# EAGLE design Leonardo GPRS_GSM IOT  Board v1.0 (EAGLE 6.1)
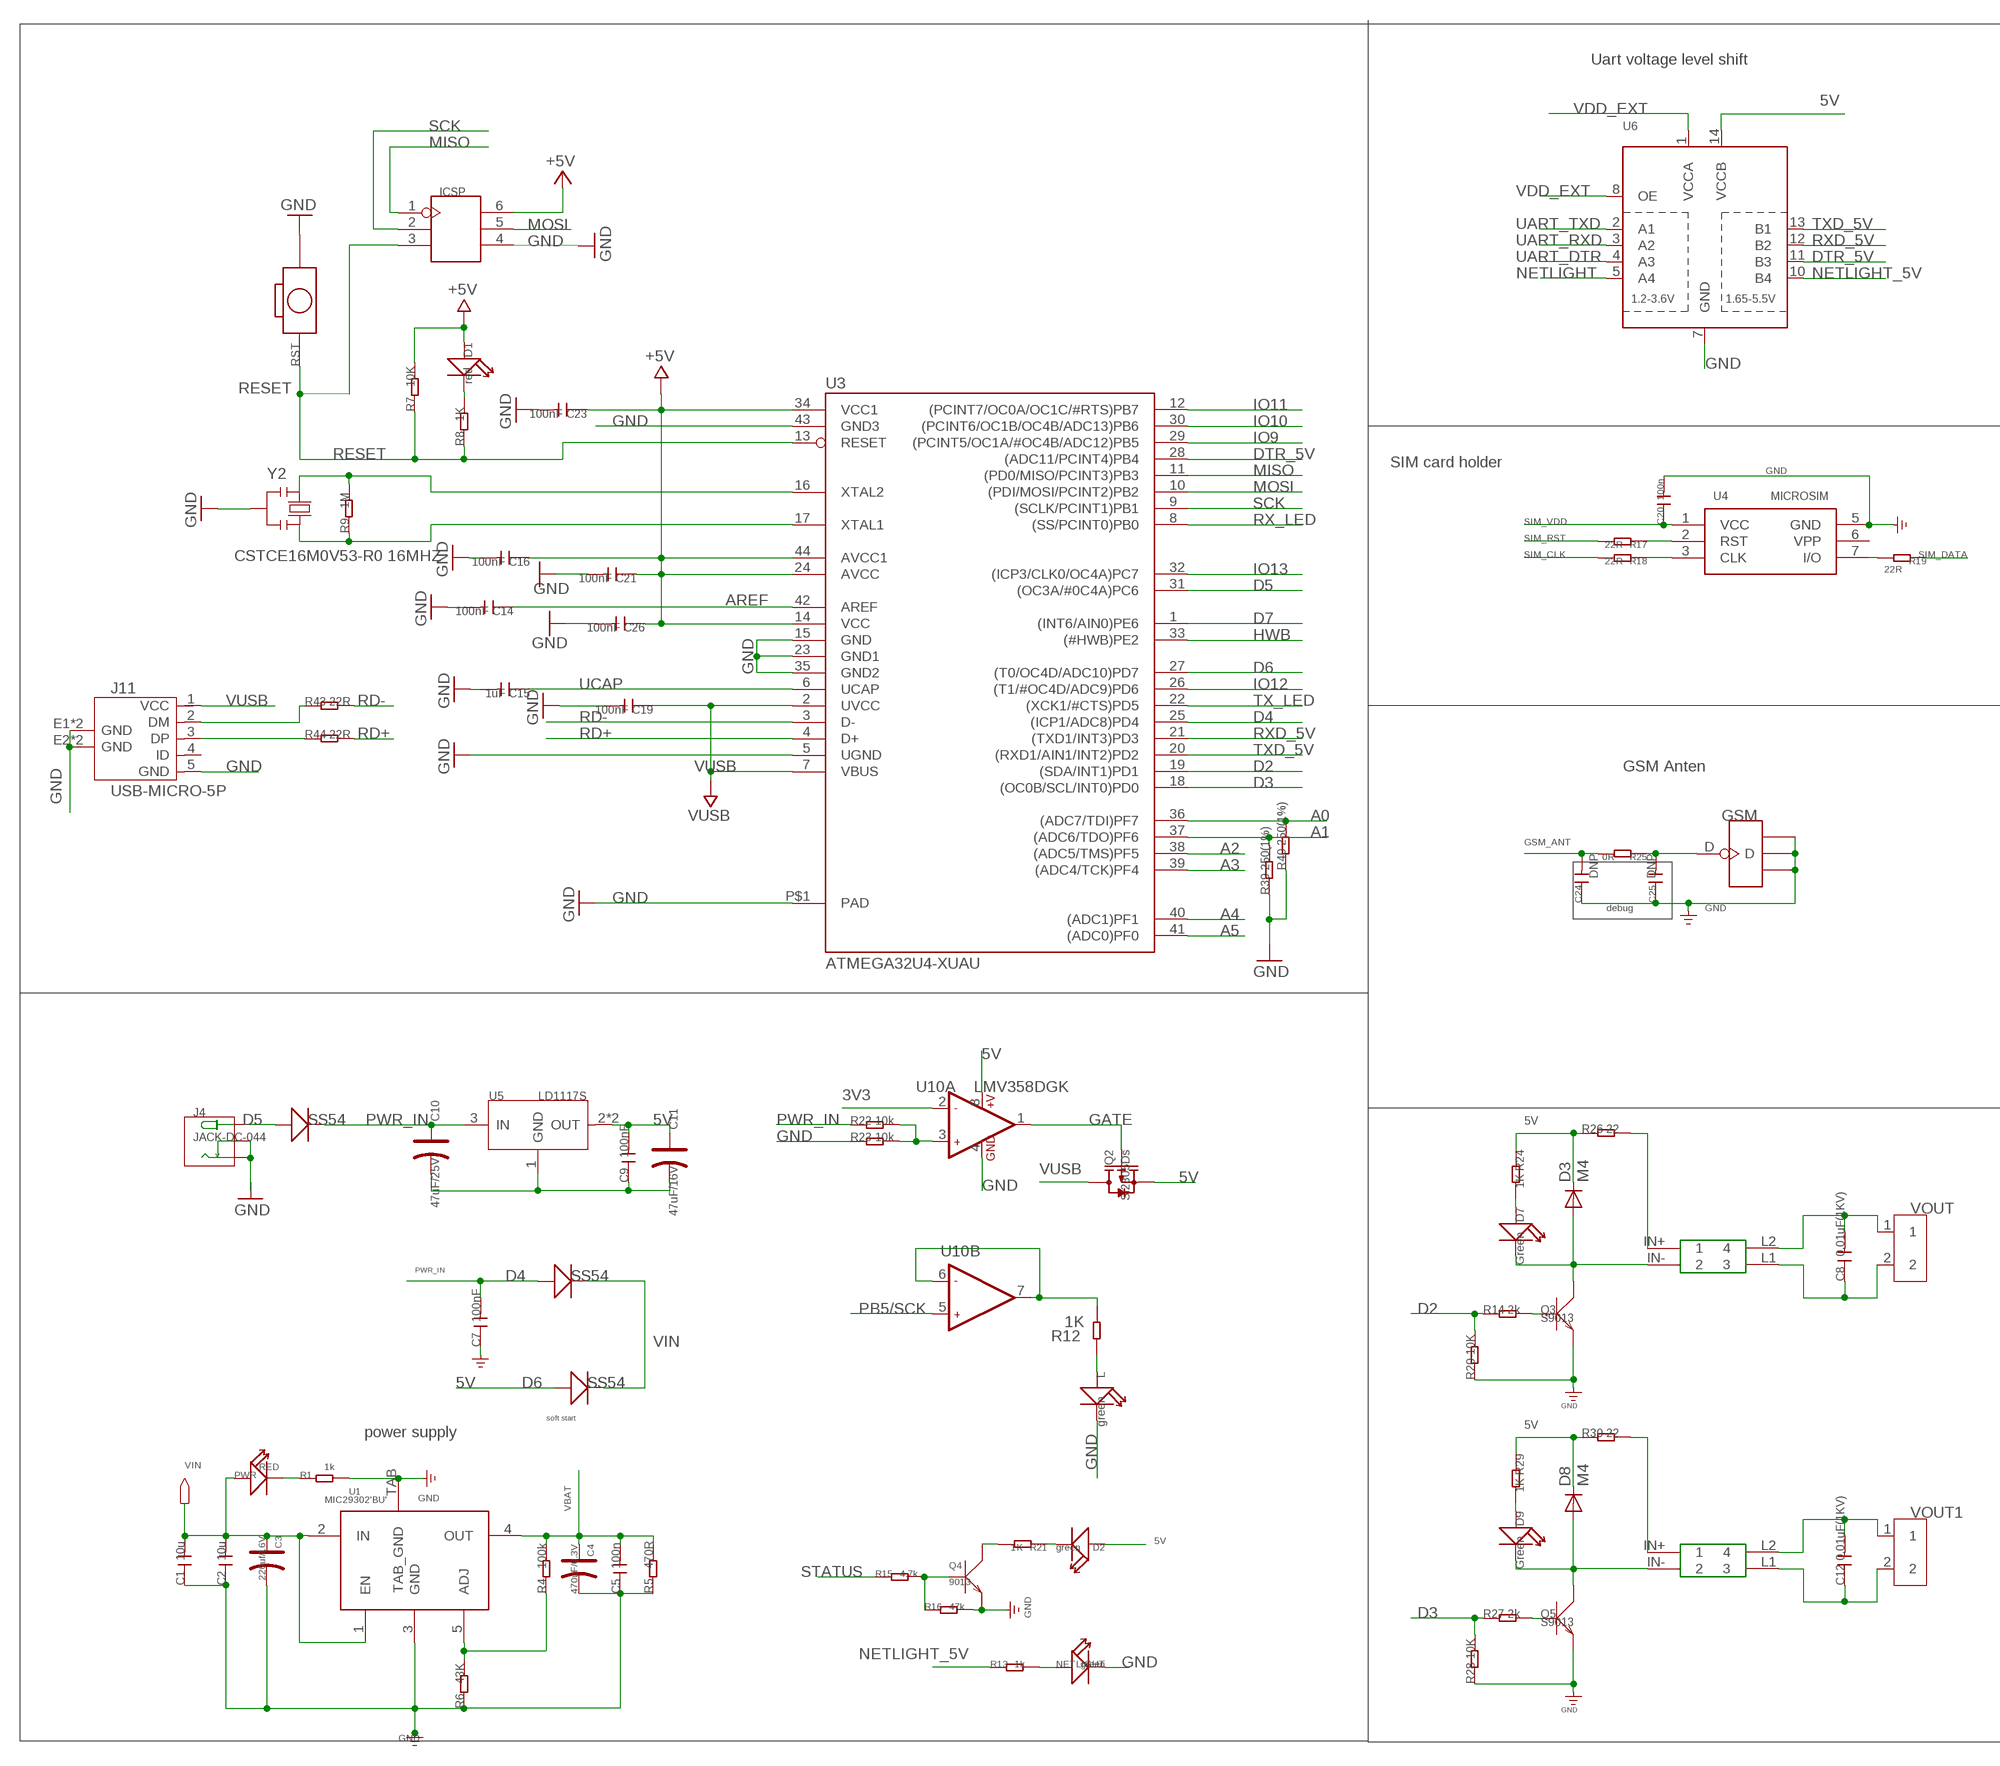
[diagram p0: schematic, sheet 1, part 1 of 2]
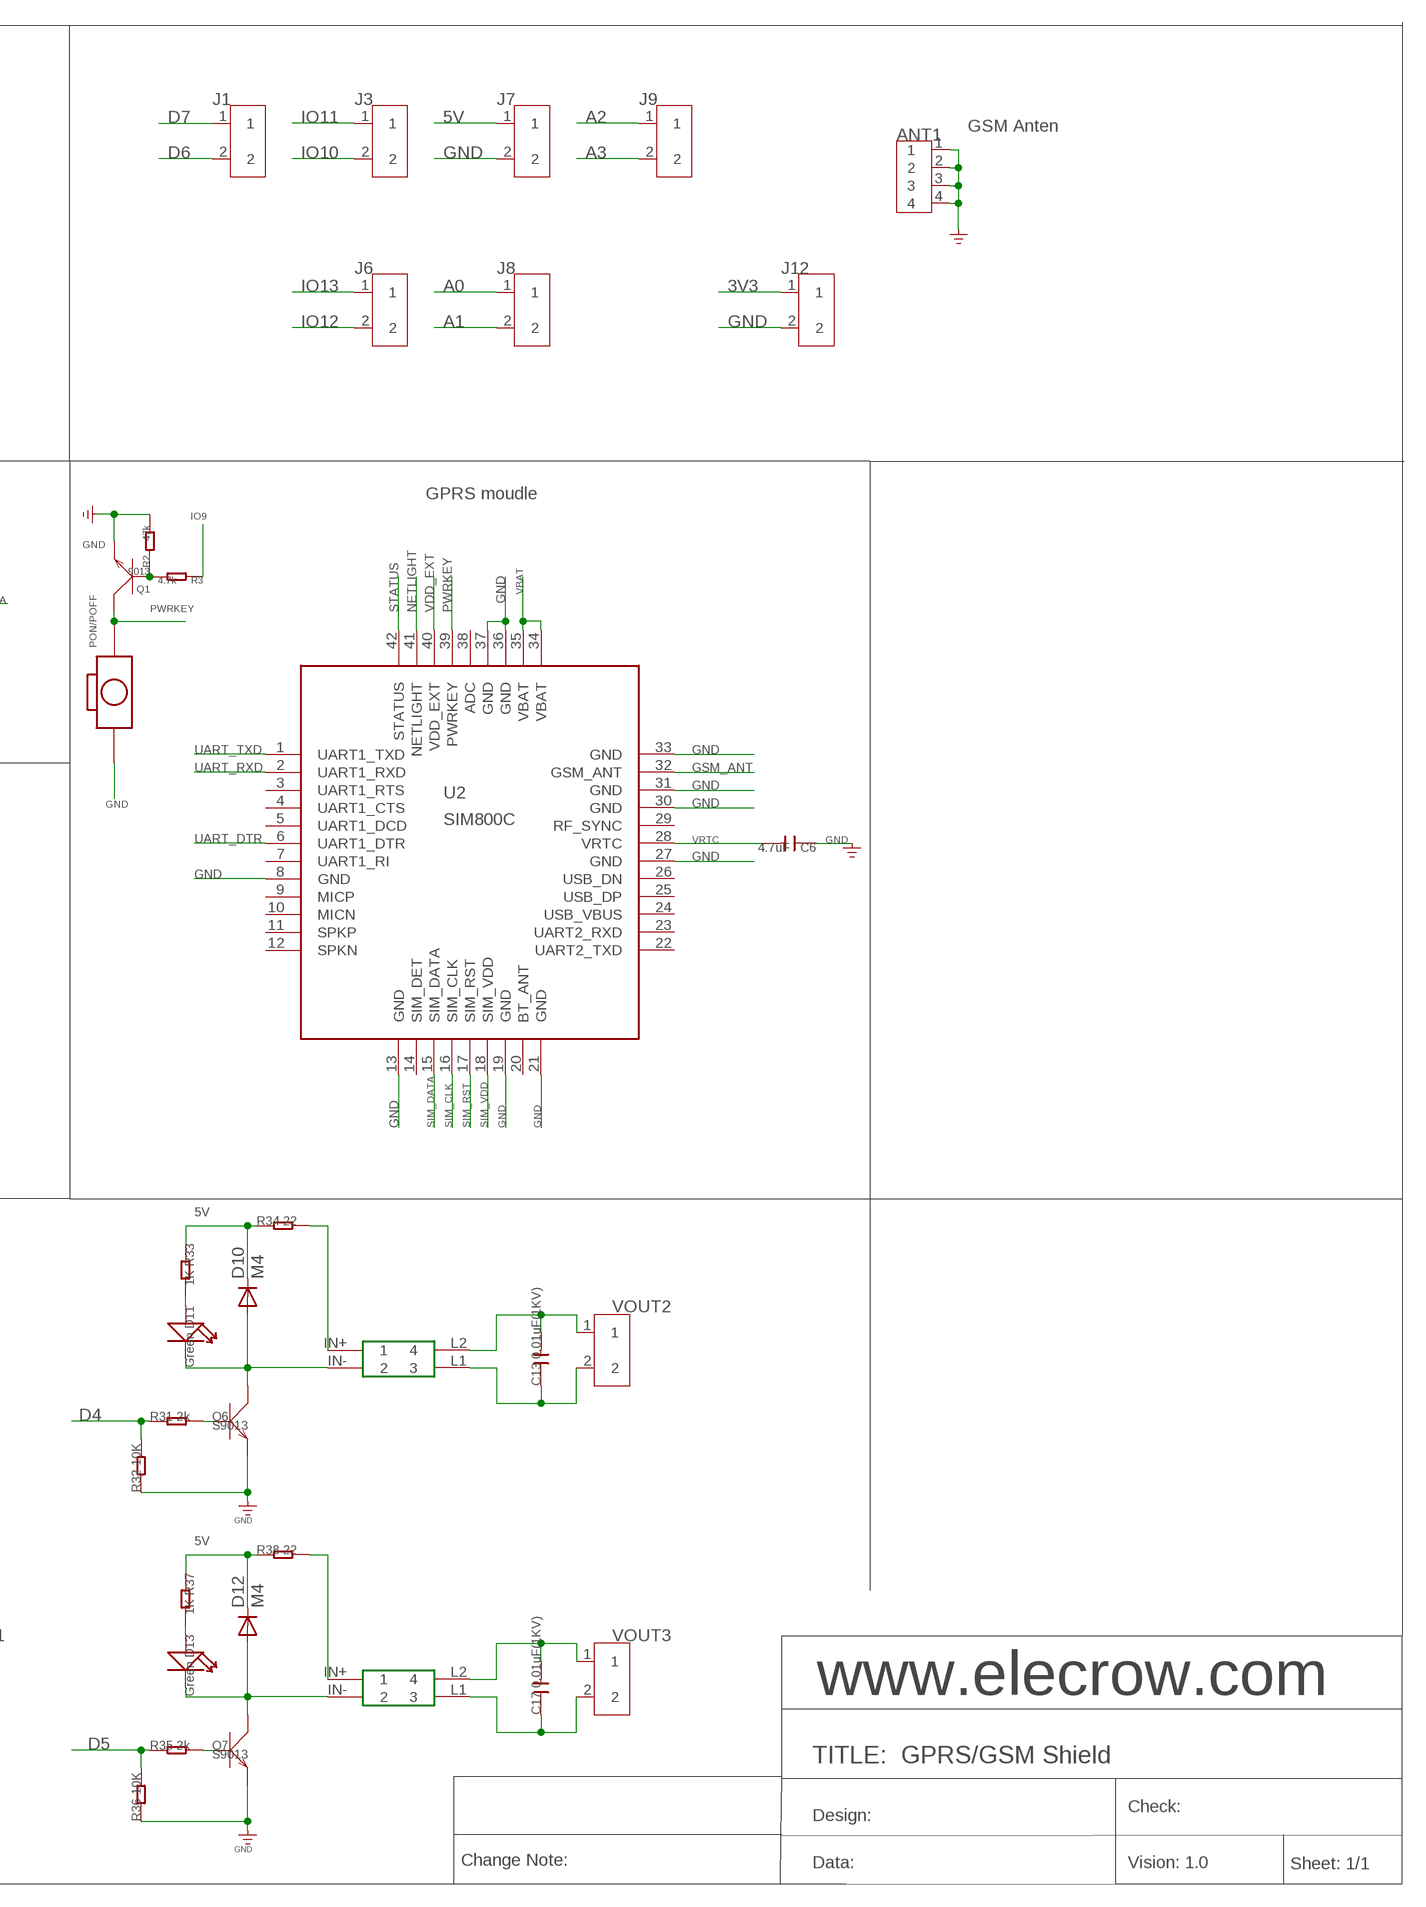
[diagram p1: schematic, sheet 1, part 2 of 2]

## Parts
ANT1  ANTENNA-SMA-IPX  [SMA-TO-IPX]
C1  10u  C-0603  [C0603]
C2  10u  C-0603  [C0603]
C3  220uf/16V  006-CAP_AVX_D  [AVX_D]
C4  470uF/6.3V  006-CAP_AVX_D  [AVX_D]
C5  100n  C-0603  [C0603]
C6  4.7uF  C-0805  [C0805]
C7  100nF  C-0603  [C0603]
C8  0.01uF(1KV)  C-1206  [C1206]
C9  100nF  C-0603  [C0603]
C10  47uF/25V  CAP-AVX-C  [AVX-C]
C11  47uF/16V  CAP-AVX-A  [AVX-A]
C12  0.01uF(1KV)  C-1206  [C1206]
C13  0.01uF(1KV)  C-1206  [C1206]
C14  100nF  C-0603  [C0603]
C15  1uF  C-0603  [C0603]
C16  100nF  C-0603  [C0603]
C17  0.01uF(1KV)  C-1206  [C1206]
C19  100nF  C-0603  [C0603]
C20  100n  C-0603  [C0603]
C21  100nF  C-0603  [C0603]
C23  100nF  C-0603  [C0603]
C24  DNP  C-0402  [C0402]
C25  DNP  C-0402  [C0402]
C26  100nF  C-0603  [C0603]
D1  red  LED'0603'  [LED-0603]
D2  green  LED'0603'  [LED-0603]
D3  M4  DIODE-DO-214AC  [DO-214AC]
D4  SS54  D'MBRS240LT3'  [SMB]
D5  SS54  D'MBRS240LT3'  [SMB]
D6  SS54  D'MBRS240LT3'  [SMB]
D7  Green  LED'0603'  [LED-0603]
D8  M4  DIODE-DO-214AC  [DO-214AC]
D9  Green  LED'0603'  [LED-0603]
D10  M4  DIODE-DO-214AC  [DO-214AC]
D11  Green  LED'0603'  [LED-0603]
D12  M4  DIODE-DO-214AC  [DO-214AC]
D13  Green  LED'0603'  [LED-0603]
GSM  ANTENNA-U-FL  [4P-U-FL]
ICSP  HEADER-2X3P-2.0  [2X3P-2.0]
J1  SCREW-TERMINAL-2P'5.0'  [2P-5.0]
J3  SCREW-TERMINAL-2P'5.0'  [2P-5.0]
J4  JACK-DC-044  [DC-404]
J6  SCREW-TERMINAL-2P'5.0'  [2P-5.0]
J7  SCREW-TERMINAL-2P'5.0'  [2P-5.0]
J8  SCREW-TERMINAL-2P'5.0'  [2P-5.0]
J9  SCREW-TERMINAL-2P'5.0'  [2P-5.0]
J11  USB-MICRO-5P  [MICRO-USB-5P]
J12  SCREW-TERMINAL-2P'5.0'  [2P-5.0]
L  green  LED'0603'  [LED-0603]
NETLIGHT  green  LED'0603'  [LED-0603]
PON/POFF  BOTTON_1_DP  [BTN_5.0_RST]
PWR  RED  007-LED0603  [D0603]
Q1  9013  TRANSISTOR-NPN-SOT23  [SOT23]
Q2  Si2305Ds  MOSFET-P'SI2323CDS/SI2305DS<BR>'  [SOT23@2]
Q3  S9013  TRANSISTOR-NPN-SOT23  [SOT23]
Q4  9013  TRANSISTOR-NPN-SOT23  [SOT23]
Q5  S9013  TRANSISTOR-NPN-SOT23  [SOT23]
Q6  S9013  TRANSISTOR-NPN-SOT23  [SOT23]
Q7  S9013  TRANSISTOR-NPN-SOT23  [SOT23]
R1  1k  R-0603  [R0603]
R2  47k  R-0603  [R0603]
R3  4.7k  R-0603  [R0603]
R4  100k  R-0603  [R0603]
R5  470R  R-0603  [R0603]
R6  43K  R-0603  [R0603]
R7  10K  R-0603  [R0603]
R8  1K  R-0603  [R0603]
R9  1M  R-0603  [R0603]
R12  1K  R-0603  [R0603]
R13  1k  R-0603  [R0603]
R14  2k  R-0603  [R0603]
R15  4.7k  R-0603  [R0603]
R16  47k  R-0603  [R0603]
R17  22R  R-0603  [R0603]
R18  22R  R-0603  [R0603]
R19  22R  R-0603  [R0603]
R20  10K  R-0603  [R0603]
R21  1K  R-0603  [R0603]
R22  10k  R-0603  [R0603]
R23  10k  R-0603  [R0603]
R24  1K  R-0603  [R0603]
R25  0R  R-0402  [R0402]
R26  22  R-0603  [R0603]
R27  2k  R-0603  [R0603]
R28  10K  R-0603  [R0603]
R29  1K  R-0603  [R0603]
R30  22  R-0603  [R0603]
R31  2k  R-0603  [R0603]
R32  10K  R-0603  [R0603]
R33  1K  R-0603  [R0603]
R34  22  R-0603  [R0603]
R35  2k  R-0603  [R0603]
R36  10K  R-0603  [R0603]
R37  1K  R-0603  [R0603]
R38  22  R-0603  [R0603]
R39  250(1%)  R-0603  [R0603]
R40  250(1%)  R-0603  [R0603]
R43  22R  R-0603  [R0603]
R44  22R  R-0603  [R0603]
RST  BOTTON-2P-90D  [2P-7.62X3.56-90D]
U1  MIC29302'BU'  [TO-263]
U2  SIM800C  [SIM800C]
U3  ATMEGA32U4-XUAU  [TQFP44-PAD]
U4  MICROSIM  [MICROSIM]
U5  LD1117S  [SOT-223]
U6  TXB0104PWR  [TSSOP14]
U10  LMV358DGK  [MSOP8]
U$5  G3MB-202(RELAY)  [G3MB-202(RELAY)]
U$8  G3MB-202(RELAY)  [G3MB-202(RELAY)]
U$10  G3MB-202(RELAY)  [G3MB-202(RELAY)]
U$12  G3MB-202(RELAY)  [G3MB-202(RELAY)]
VOUT  SCREW-TERMINAL-2P'5.0'  [2P-5.0]
VOUT1  SCREW-TERMINAL-2P'5.0'  [2P-5.0]
VOUT2  SCREW-TERMINAL-2P'5.0'  [2P-5.0]
VOUT3  SCREW-TERMINAL-2P'5.0'  [2P-5.0]
Y2  CSTCE16M0V53-R0 16MHZ  RESONATORMU  [RESONATOR]

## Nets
3V3: J12.1 U10.2(A:-IN1)
5V: C9.2 C11.+ C16.1 C21.1 C23.1 C26.1 D2.+ D3.C D6.+ D8.C D10.C D12.C ICSP.6 J7.1 Q2.2(S) R24.1 R26.1 R29.1 R30.1 R33.1 R34.1 R37.1 R38.1 U3.14(VCC) U3.24(AVCC) U3.34(VCC1) U3.44(AVCC1) U5.2(OUT) U5.TER(OUT) U6.14(VCCB) U10.8(A:+V) ; supply symbol labelled +5V
+5V: D1.+ R7.2
A0: J8.1 R40.2 U3.36((ADC7/TDI)PF7)
A1: J8.2 R39.2 U3.37((ADC6/TDO)PF6)
A2: J9.1 U3.38((ADC5/TMS)PF5)
A3: J9.2 U3.39((ADC4/TCK)PF4)
A4: U3.40((ADC1)PF1)
A5: U3.41((ADC0)PF0)
AREF: C14.1 U3.42(AREF)
D2: R14.1 R20.2 U3.19((SDA/INT1)PD1)
D3: R27.1 R28.2 U3.18((OC0B/SCL/INT0)PD0)
D4: R31.1 R32.2 U3.25((ICP1/ADC8)PD4)
D5: R35.1 R36.2 U3.31((OC3A/#0C4A)PC6)
D6: J1.2 U3.27((T0/OC4D/ADC10)PD7)
D7: J1.1 U3.1((INT6/AIN0)PE6)
D+1: J11.3(DP) R44.1
D-1: J11.2(DM) R43.1
DTR_5V: U3.28((ADC11/PCINT4)PB4) U6.11(B3)
GATE: Q2.1(G) U10.1(A:OUT1)
GND: ANT1.1 ANT1.2 ANT1.3 ANT1.4 C1.1 C2.1 C3.- C4.- C5.1 C6.1 C7.1 C9.1 C10.- C11.- C14.2 C15.2 C16.2 C19.2 C20.2 C21.2 C23.2 C24.1 C25.1 C26.2 GSM.GND1 GSM.GND2 GSM.GND3 ICSP.4 J4.- J4.CDN J7.2 J11.5(GND) J11.E1(GND) J11.E2(GND) J11.P1(GND) J11.P2(GND) J12.2 L.- NETLIGHT.- PON/POFF.P$1 Q1.2(E) Q3.2(E) Q4.2(E) Q5.2(E) Q6.2(E) Q7.2(E) R1.2 R2.2 R5.1 R6.1 R16.2 R20.1 R23.1 R28.1 R32.1 R36.1 R39.1 R40.1 RST.P$2 U1.3(GND) U1.TAB(TAB_GND) U2.8(GND) U2.13(GND) U2.19(GND) U2.21(GND) U2.27(GND) U2.30(GND) U2.31(GND) U2.33(GND) U2.36(GND) U2.37(GND) U3.5(UGND) U3.15(GND) U3.23(GND1) U3.35(GND2) U3.43(GND3) U3.P$1(PAD) U4.5(GND) U5.1(GND) U6.7(GND) U10.4(A:GND) Y2.2
GSM_ANT: C24.2 R25.2 U2.32(GSM_ANT)
HWB: U3.33((#HWB)PE2)
IO9: R3.1 U3.29((PCINT5/OC1A/#OC4B/ADC12)PB5)
IO10: J3.2 U3.30((PCINT6/OC1B/OC4B/ADC13)PB6)
IO11: J3.1 U3.12((PCINT7/OC0A/OC1C/#RTS)PB7)
IO12: J6.2 U3.26((T1/#OC4D/ADC9)PD6)
IO13: J6.1 U3.32((ICP3/CLK0/OC4A)PC7)
MISO: ICSP.1 U3.11((PD0/MISO/PCINT3)PB3)
MOSI: ICSP.5 U3.10((PDI/MOSI/PCINT2)PB2)
N$1: R19.2 U4.7(I/O)
N$2: R4.1 R6.2 U1.5(ADJ)
N$3: Q3.1(B) R14.2
N$4: D5.+ J4.+
N$5: R18.1 U4.3(CLK)
N$6: R17.1 U4.2(RST)
N$7: NETLIGHT.+ R13.2
N$8: D3.A D7.- Q3.3(C) U$5.IN-
N$9: L.+ R12.2
N$10: Q6.1(B) R31.2
N$11: R12.1 U10.6(B:-IN2) U10.7(B:OUT2)
N$12: D7.+ R24.2
N$13: D10.A D11.- Q6.3(C) U$10.IN-
N$14: R22.2 R23.2 U10.3(A:+IN1)
N$15: D1.- R8.2
N$16: Q4.3(C) R21.2
N$17: D2.- R21.1
N$18: Q4.1(B) R15.2 R16.1
N$19: R26.2 U$5.IN+
N$20: C8.2 U$5.L2 VOUT.1
N$21: C8.1 U$5.L1 VOUT.2
N$22: Q5.1(B) R27.2
N$23: D8.A D9.- Q5.3(C) U$8.IN-
N$24: D9.+ R29.2
N$25: C25.2 GSM.D R25.1
N$26: R30.2 U$8.IN+
N$27: C12.2 U$8.L2 VOUT1.1
N$28: C12.1 U$8.L1 VOUT1.2
N$29: D11.+ R33.2
N$30: R34.2 U$10.IN+
N$31: C13.2 U$10.L2 VOUT2.1
N$32: C13.1 U$10.L1 VOUT2.2
N$33: Q7.1(B) R35.2
N$34: D12.A D13.- Q7.3(C) U$12.IN-
N$35: D13.+ R37.2
N$36: Q1.1(B) R2.1 R3.2
N$37: R38.2 U$12.IN+
N$38: C17.2 U$12.L2 VOUT3.1
N$39: C17.1 U$12.L1 VOUT3.2
N$53: PWR.- R1.1
NETLIGHT: U2.41(NETLIGHT) U6.5(A4)
NETLIGHT_5V: R13.1 U6.10(B4)
PB5/SCK: U10.5(B:+IN2)
PWR_IN: C7.2 C10.+ D4.+ D5.- R22.1 U5.3(IN)
PWRKEY: PON/POFF.P$2 Q1.3(C) U2.39(PWRKEY)
RD+: R44.2 U3.4(D+)
RD-: R43.2 U3.3(D-)
RESET: ICSP.3 R7.1 R8.1 RST.P$1 U3.13(RESET)
RX_LED: U3.8((SS/PCINT0)PB0)
RXD_5V: U3.21((TXD1/INT3)PD3) U6.12(B2)
SCK: ICSP.2 U3.9((SCLK/PCINT1)PB1)
SIM_CLK: R18.2 U2.16(SIM_CLK)
SIM_DATA: R19.1 U2.15(SIM_DATA)
SIM_RST: R17.2 U2.17(SIM_RST)
SIM_VDD: C20.1 U2.18(SIM_VDD) U4.1(VCC)
STATUS: R15.1 U2.42(STATUS)
TX_LED: U3.22((XCK1/#CTS)PD5)
TXD_5V: U3.20((RXD1/AIN1/INT2)PD2) U6.13(B1)
UART_DTR: U2.6(UART1_DTR) U6.4(A3)
UART_RXD: U2.2(UART1_RXD) U6.3(A2)
UART_TXD: U2.1(UART1_TXD) U6.2(A1)
UCAP: C15.1 U3.6(UCAP)
VBAT: C4.+ C5.2 R4.2 R5.2 U1.4(OUT) U2.34(VBAT) U2.35(VBAT)
VDD_EXT: U2.40(VDD_EXT) U6.1(VCCA) U6.8(OE)
VIN: C1.2 C2.2 C3.+ D4.- D6.- PWR.+ U1.1(EN) U1.2(IN)
VRTC: C6.2 U2.28(VRTC)
VUSB: C19.1 J11.1(VCC) Q2.3(D) U3.2(UVCC) U3.7(VBUS)
XTAL3: R9.2 U3.16(XTAL2) Y2.1
XTAL4: R9.1 U3.17(XTAL1) Y2.3
Unconnected: J11.4(ID) U2.3(UART1_RTS) U2.4(UART1_CTS) U2.5(UART1_DCD) U2.7(UART1_RI) U2.9(MICP) U2.10(MICN) U2.11(SPKP) U2.12(SPKN) U2.14(SIM_DET) U2.20(BT_ANT) U2.22(UART2_TXD) U2.23(UART2_RXD) U2.24(USB_VBUS) U2.25(USB_DP) U2.26(USB_DN) U2.29(RF_SYNC) U2.38(ADC) U4.6(VPP)

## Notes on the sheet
- Uart voltage level shift
- GSM Anten
- GPRS moudle
- SIM card holder
- GSM Anten
- debug
- soft start
- power supply
- www.elecrow.com
- TITLE:  GPRS/GSM Shield
- Check:
- Design:
- Change Note: | Data: | Vision: 1.0 | Sheet: 1/1

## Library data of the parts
ANT1 = Connector:ANTENNA-SMA-IPX
C1 C2 C5-C9 C12-C17 C19-C21 C23-C26 = Discrete:C*: Ceramic Capacitors
C3 C4 = Discrete:006-CAP*: Electrolytic Capacitors,Tantalum Capacitors and Super Capacitors
C10 C11 = Discrete:CAP*: Electrolytic Capacitors,Tantalum Capacitors and Super Capacitors
D1 D2 D7 D9 D11 D13 L NETLIGHT = Discrete:LED*
D3 D8 D10 D12 = diode:DIODE-: DIODE
D4-D6 = Discrete:D*
GSM = Connector:ANTENNA-U-FL
ICSP = Connector:HEADER-2X3P
J1 J3 J6-J9 J12 VOUT VOUT1-VOUT3 = Connector:SCREW-TERMINAL-2P
J4 = Connector:JACK-DC-044
J11 = Connector:USB-MICRO-5P
PON/POFF = CPT_SMD:BOTTON_1
PWR = Discrete:007-LED*
Q1 Q3-Q7 = Discrete:TRANSISTOR-NPN*: NPN audion
Q2 = Discrete:MOSFET-P
R1-R9 R12-R40 R43 R44 = Discrete:R*
RST = Discrete:BOTTON-2P
U1 = ICs_v54:MIC29302
U2 = moudle:SIM800C
U3 = SmartPrj:ATMEGA32U4-XU
U4 = Connector:MICROSIM
U5 = IC:LD1117: Low Drop Fixed And Adjustable Positive Voltage Regulators http://www.datasheetcatalog.org/datasheet/SGSThomsonMicroelectronics/mXuqtqv.pdf
U6 = adafruit:TXB0104PWR: 4-Bit Bi-Directional Level Shifter 1.2V-3.6V (VCCA) to 1.65V-5.5V (VCCB) bi-directional level shifter with auto direction sensing. Max data rate - VCCA 1.8V: 20Mbps (50ns), VCCA 3.3V: 100Mbps (10ns) Digikey: 296-21929-1-ND
U10 = IC:LMV358: General purpose LOW Voltage, Rail-to-Rail Output Amplifiers http://www.fairchildsemi.com/ds/LM/LMV358.pdf
U$5 U$8 U$10 U$12 = G3MB-202(relay):G3MB-202(RELAY)
Y2 = SmartPrj:RESONATOR

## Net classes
0 default: width 0.152 mm, drill 0.152 mm, clearance 0.152 mm
3 usbvcc: width 0.508 mm, drill 0.61 mm, clearance 0.254 mm
4 aref: width 0.254 mm, drill 0.61 mm, clearance 0.254 mm

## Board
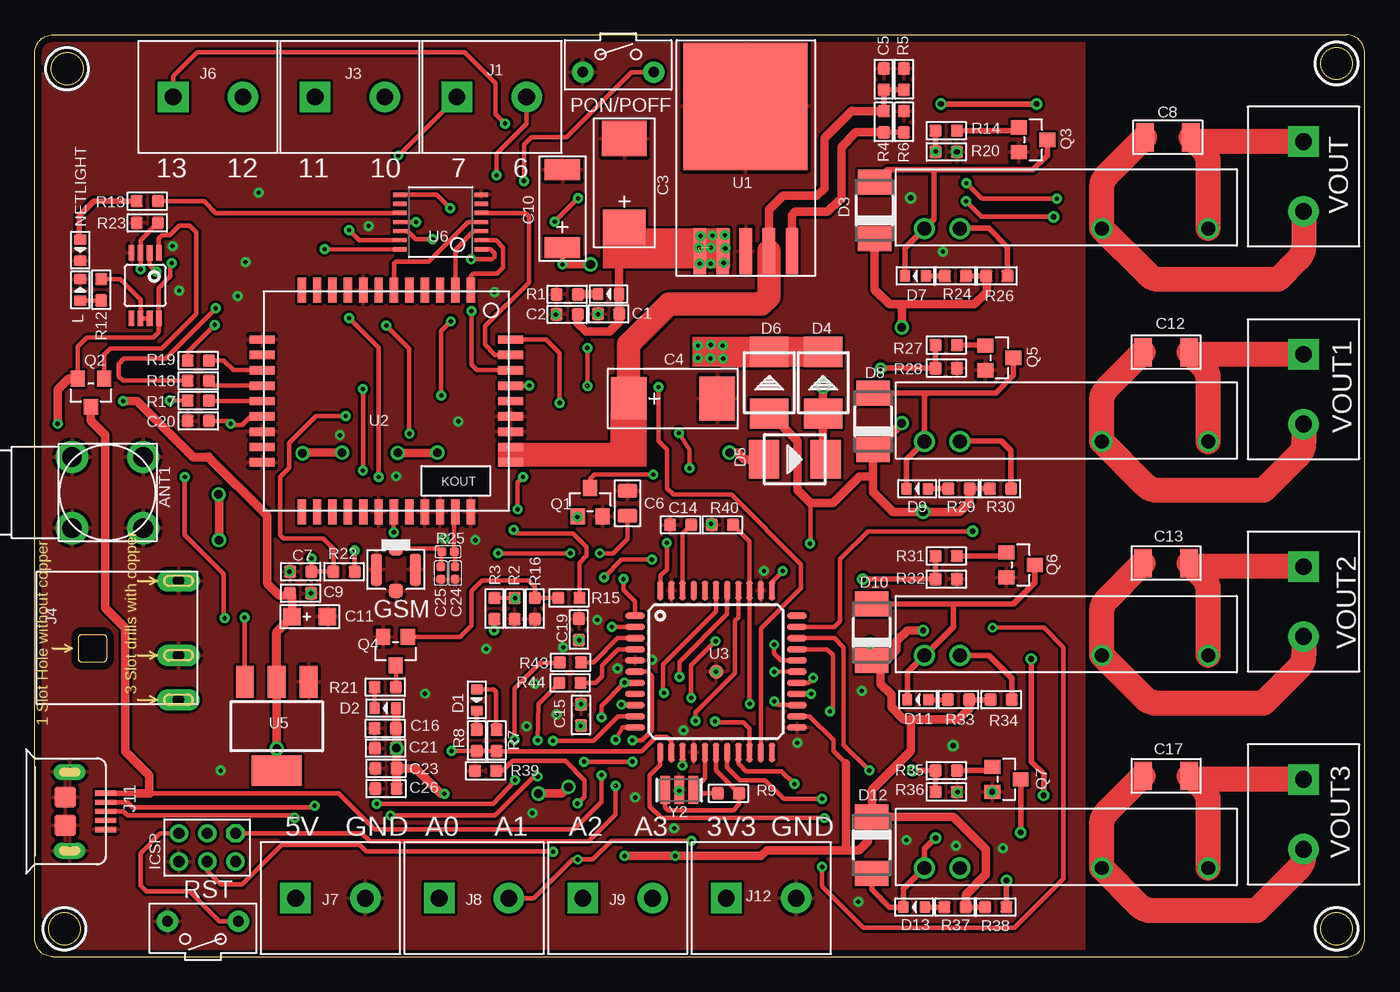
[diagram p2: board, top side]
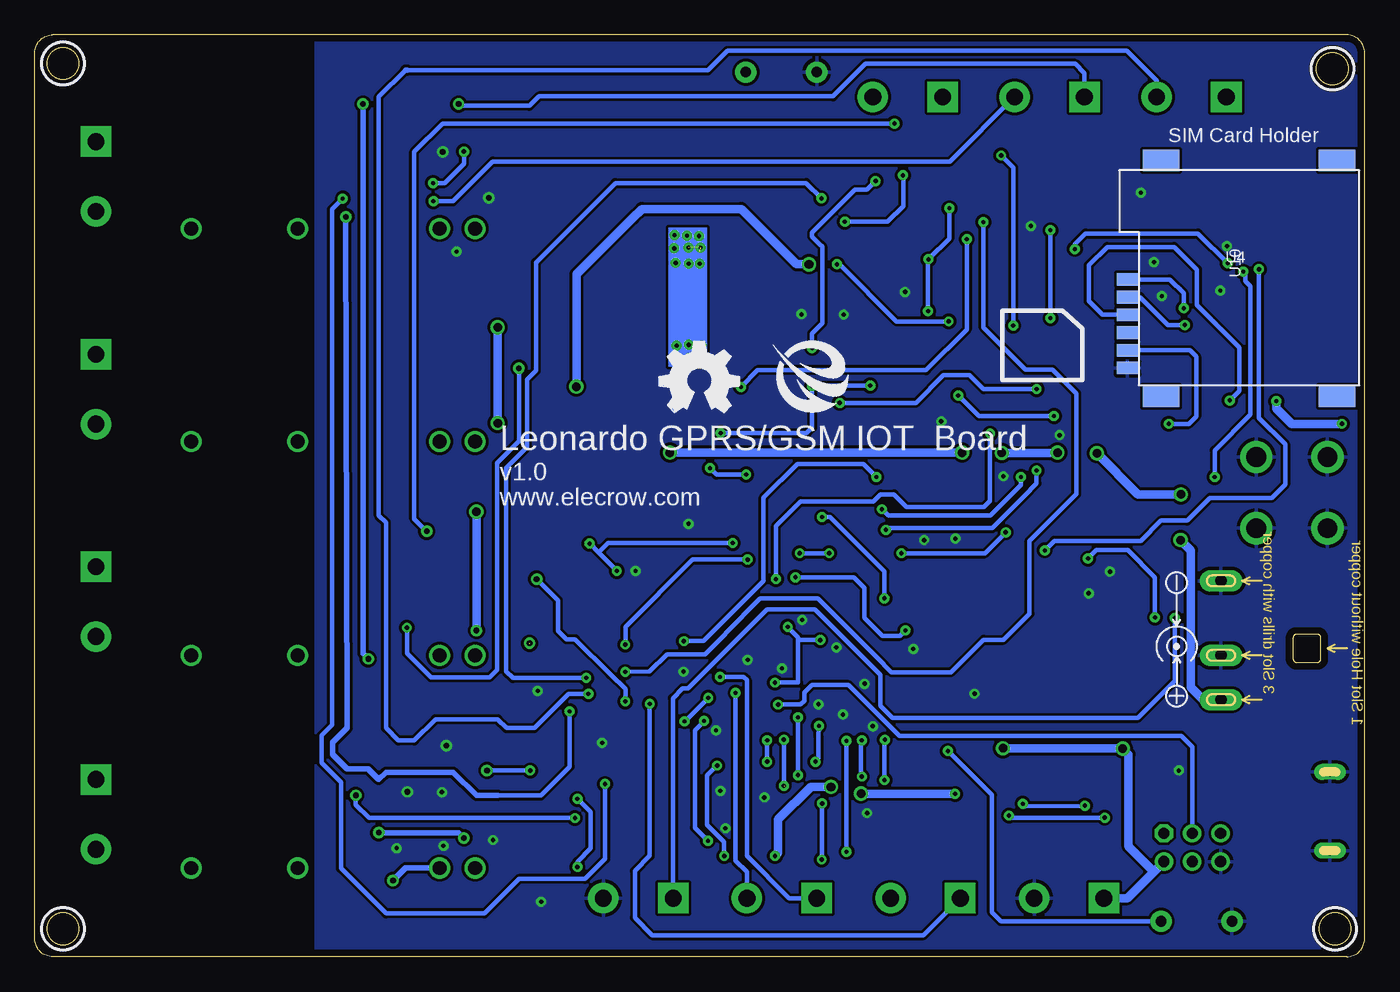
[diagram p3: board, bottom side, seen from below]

Size 95.25 x 66.04 mm. Coordinates in mm from the lower left corner, seen from the top.
Outline: 1.27,0 93.98,0 arc90 95.25,1.27 95.25,64.77 arc90 93.98,66.04 1.27,66.04 arc90 0,64.77 0,1.27 arc90 1.27,0
Outline: circle at 2.13,2 radius 1.14
Outline: circle at 2.13,2 radius 1.14
Outline: circle at 93.24,64 radius 1.14
Outline: circle at 93.24,64 radius 1.14
Outline: circle at 2.31,63.62 radius 1.14
Outline: circle at 2.31,63.62 radius 1.14
Outline: circle at 93.24,2 radius 1.14
Outline: circle at 93.24,2 radius 1.14
Copper layers (1*16): Top 0.035mm / dielectric 1.5mm / Bottom 0.035mm
Design rules: minimum track width 10mil, minimum drill 12mil, track to track 8mil, track to pad 8mil, pad to pad 8mil, via to via 8mil, smd to smd 0mil, copper to edge 20mil, drill to drill 8mil, minimum pad ring 10mil, minimum via ring 8mil, stop-mask expansion 4mil, vias tented up to drill 100mil, thermal gap 10mil
tRestrict: area 0.6,0.5 to 3.7,3.5; area 91.7,62.5 to 94.8,65.5; area 0.8,62.1 to 3.8,65.1; area 91.7,0.5 to 94.8,3.5; 1 lines
bRestrict: area 0.6,0.5 to 3.7,3.5; area 91.7,62.5 to 94.8,65.5; area 0.8,62.1 to 3.8,65.1; area 91.7,0.5 to 94.8,3.5

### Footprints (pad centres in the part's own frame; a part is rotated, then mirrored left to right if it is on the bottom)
SMA-TO-IPX = drill 1.4 pad 2.3: 1 -2.55,2.55; 2 2.55,2.55; 3 2.55,-2.55; 4 -2.55,-2.55
C0603 = smd 0.889 x 0.889: 1 -0.762,0; 2 0.762,0
AVX_D = smd 2.54 x 3.048: + -3.175,0 | smd 2.54 x 3.175: - 3.175,0
C0805 = smd 1.016 x 1.397: 1 -0.889,0; 2 0.889,0
C1206 = smd 1.27 x 2.032: 1 -1.651,0; 2 1.651,0
AVX-C = smd 1.524 x 2.54: + -2.794,0; - 2.794,0
AVX-A = smd 1.27 x 1.27: + -1.27,0; - 1.27,0
C0402 = smd 0.635 x 0.635: 1 -0.445,0; 2 0.445,0
LED-0603 = smd 0.762 x 0.889: + -0.762,0; - 0.762,0
DO-214AC = smd 1.8 x 2.4: A 2.025,0; C -2.025,0
SMB = smd 2.159 x 2.743: + -2.21,0; - 2.21,0
4P-U-FL = smd 1.016 x 1.016: D -1.524,0; GND3 1.524,0 | smd 2.286 x 0.762: GND1 0,1.397; GND2 0,-1.397
2X3P-2.0 = drill 0.813 pad 1.27 octagon: 1 -1.016,2.032 | drill 0.813 pad 1.27: 2 -1.016,0; 3 -1.016,-2.032; 4 1.016,-2.032; 5 1.016,0; 6 1.016,2.032
2P-5.0 = drill 1.2 pad 2.184 square: 1 0,0 | drill 1.2 pad 2.184: 2 5,0
DC-404 = drill 0.813 pad 1.524 long: + 3.175,10.16; - -5.334,10.16; CDN 0,10.16
MICRO-USB-5P = smd 0.38 x 1.52: 1 -1.3,0; 2 -0.65,0; 3 0,0; 4 0.65,0; 5 1.3,0 | smd 1.524 x 1.524: E1 -1.016,-2.921; E2 1.016,-2.921 | drill 0.635 pad 1.143 long: P1 -2.819,-2.591; P2 2.819,-2.591
BTN_5.0_RST = drill 0.762 pad 1.524: P$1 0,2.54; P$2 0,-2.54
D0603 = smd 0.762 x 0.889: + -0.762,0; - 0.762,0
SOT23 = smd 1.016 x 1.143: 1 -0.889,-1.016; 2 0.889,-1.016; 3 0,1.016
SOT23@2 = smd 1.016 x 1.143: 1 -0.95,-1.016; 2 0.95,-1.016; 3 0,1.016
R0603 = smd 0.889 x 0.889: 1 -0.762,0; 2 0.762,0
R0402 = smd 0.635 x 0.635: 1 -0.445,0; 2 0.445,0
2P-7.62X3.56-90D = drill 0.762 pad 1.524: P$1 0,2.54; P$2 0,-2.54
TO-263 = smd 3.302 x 0.889: 1 3.302,-3.302; 2 3.302,-1.651; 3 3.302,0; 4 3.302,1.651; 5 3.302,3.302 | smd 9.12 x 8.89: TAB -7.071,-0.03
SIM800C = smd 1.8 x 0.6: 1 -7.95,6.05; 2 -7.95,4.95; 3 -7.95,3.85; 4 -7.95,2.75; 5 -7.95,1.65; 6 -7.95,0.55; 7 -7.95,-0.55; 8 -7.95,-1.65; 9 -7.95,-2.75; 10 -7.95,-3.85; 11 -7.95,-4.95; 12 -7.95,-6.05; 22 7.95,-6.05; 23 7.95,-4.95; 24 7.95,-3.85; 25 7.95,-2.75; 26 7.95,-1.65; 27 7.95,-0.55; 28 7.95,0.55; 29 7.95,1.65; 30 7.95,2.75; 31 7.95,3.85; 32 7.95,4.95; 33 7.95,6.05 | smd 0.6 x 1.8: 13 -4.4,-8.9; 14 -3.3,-8.9; 15 -2.2,-8.9; 16 -1.1,-8.9; 17 0,-8.9; 18 1.1,-8.9; 19 2.2,-8.9; 20 3.3,-8.9; 21 4.4,-8.9; 34 4.4,8.9; 35 3.3,8.9; 36 2.2,8.9; 37 1.1,8.9; 38 0,8.9; 39 -1.1,8.9; 40 -2.2,8.9; 41 -3.3,8.9; 42 -4.4,8.9
TQFP44-PAD = smd 1.4 x 0.45: 1 -5.8,4; 2 -5.8,3.2; 3 -5.8,2.4; 4 -5.8,1.6; 5 -5.8,0.8; 6 -5.8,0; 7 -5.8,-0.8; 8 -5.8,-1.6; 9 -5.8,-2.4; 10 -5.8,-3.2; 11 -5.8,-4; 23 5.8,-4; 24 5.8,-3.2; 25 5.8,-2.4; 26 5.8,-1.6; 27 5.8,-0.8; 28 5.8,0; 29 5.8,0.8; 30 5.8,1.6; 31 5.8,2.4; 32 5.8,3.2; 33 5.8,4 | smd 0.45 x 1.4: 12 -4,-5.8; 13 -3.2,-5.8; 14 -2.4,-5.8; 15 -1.6,-5.8; 16 -0.8,-5.8; 17 0,-5.8; 18 0.8,-5.8; 19 1.6,-5.8; 20 2.4,-5.8; 21 3.2,-5.8; 22 4,-5.8; 34 4,5.8; 35 3.2,5.8; 36 2.4,5.8; 37 1.6,5.8; 38 0.8,5.8; 39 0,5.8; 40 -0.8,5.8; 41 -1.6,5.8; 42 -2.4,5.8; 43 -3.2,5.8; 44 -4,5.8 | smd 1 x 1: P$1 0,0
MICROSIM = smd 1.5 x 0.9: 1 -0.8,2.5; 2 -0.8,5.04; 3 -0.8,7.58; 5 -0.8,1.23; 6 -0.8,3.77; 7 -0.8,6.31 | smd 2.61 x 1.56: P$1 1.6,-0.8; P$2 14.2,-0.8; P$3 14.2,16.1; P$4 1.6,16.1
SOT-223 = smd 1.27 x 2.286: 1 -2.286,-3.175; 2 0,-3.175; 3 2.286,-3.175 | smd 3.556 x 2.159: TER 0,3.175
TSSOP14 = smd 0.305 x 0.991: 1 -1.95,-2.918; 2 -1.3,-2.918; 3 -0.65,-2.918; 4 0,-2.918; 5 0.65,-2.918; 6 1.3,-2.918; 7 1.95,-2.918; 8 1.95,2.918; 9 1.3,2.918; 10 0.65,2.918; 11 0,2.918; 12 -0.65,2.918; 13 -1.3,2.918; 14 -1.95,2.918
MSOP8 = smd 0.4 x 1.1: 1 -0.975,-2.35; 2 -0.325,-2.35; 3 0.325,-2.35; 4 0.975,-2.35; 5 0.975,2.35; 6 0.325,2.35; 7 -0.325,2.35; 8 -0.975,2.35
G3MB-202(RELAY) = drill 1: IN+ -7.62,2.54; IN- -10.16,2.54; L1 2.54,2.54; L2 10.16,2.54
RESONATOR = smd 0.7 x 2: 1 -1,0; 2 0,0; 3 1,0

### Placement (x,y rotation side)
ANT1  5.21,33.25 270 top
C1  41.1,46.05 0 top
C2  38.13,46.02 0 top
C3  42.23,55.44 90 top
C4  45.71,39.99 0 top
C5  60.81,62.87 270 top
C6  42.44,32.49 270 top
C7  19.05,27.58 0 top
C8  81.15,58.7 0 top
C9  19.02,26.04 180 top
C10  37.8,53.59 90 top
C11  19.68,24.36 0 top
C12  81.03,43.31 0 top
C13  81.03,28.19 0 top
C14  46.25,30.94 180 top
C15  39.12,17.32 90 top
C16  25.1,16.36 180 top
C17  81.03,12.95 0 top
C19  38.96,23.44 90 top
C20  11.71,38.39 180 top
C21  25.12,14.94 180 top
C23  25.15,13.49 180 top
C24  30.1,27.48 90 top
C25  29.08,27.48 90 top
C26  25.15,12.04 180 top
D1  31.65,18.39 270 top
D2  25.1,17.81 180 top
D3  60.15,53.47 90 top
D4  56.46,41.12 90 top
D5  54.43,35.64 0 top
D6  52.6,41.12 90 top
D7  63.07,48.77 180 top
D8  60.05,38.35 90 top
D9  63.2,33.53 180 top
D10  59.94,23.24 90 top
D11  63.25,18.41 180 top
D12  59.94,8 270 top
D13  62.99,3.56 180 top
GSM  25.86,27.74 270 top
ICSP  12.34,7.82 270 top
J1  30.23,61.59 0 top
J3  20.07,61.59 0 top
J4  0.13,21.59 270 top
J6  9.91,61.59 0 top
J7  18.67,4.19 0 top
J8  28.96,4.19 0 top
J9  39.24,4.19 0 top
J11  5.08,10.41 270 top
J12  49.53,4.19 0 top
L  3.25,47.78 90 top
LOGO2  LOGO-OSHW-FILLX0200-NT  [OSHW_FILLX200_NOTEXT]  50.5,38.99 0 bottom
NETLIGHT  3.25,50.62 270 top
PON/POFF  41.78,63.37 90 top
PWR  41.09,47.47 180 top
Q1  39.78,32.56 0 top
Q2  4.01,40.41 180 top
Q3  71.5,58.52 270 top
Q4  25.83,21.89 180 top
Q5  69.09,42.9 270 top
Q6  70.61,28.07 270 top
Q7  69.6,12.7 270 top
R1  38.13,47.46 180 top
R2  34.37,24.94 270 top
R3  32.92,24.94 90 top
R4  60.81,59.82 90 top
R5  62.26,62.87 270 top
R6  62.26,59.82 270 top
R7  33.07,15.49 90 top
R8  31.65,15.49 90 top
R9  49.68,11.71 180 top
R12  4.75,47.78 270 top
R13  8.05,54.13 180 top
R14  65.28,59.18 0 top
R15  38.25,25.7 180 top
R16  35.81,24.94 270 top
R17  11.71,39.84 0 top
R18  11.71,41.26 0 top
R19  11.71,42.71 180 top
R20  65.28,57.66 180 top
R21  25.1,19.3 0 top
R22  22.15,27.58 0 top
R23  8.05,52.58 0 top
R24  65.94,48.77 180 top
R25  29.59,29.01 0 top
R26  68.91,48.77 0 top
R27  65.28,43.81 0 top
R28  65.28,42.16 180 top
R29  66.19,33.53 180 top
R30  69.16,33.53 0 top
R31  65.28,28.7 0 top
R32  65.28,27.05 180 top
R33  66.17,18.41 180 top
R34  69.22,18.41 0 top
R35  65.28,13.34 0 top
R36  65.28,11.81 180 top
R37  65.91,3.56 180 top
R38  68.83,3.56 0 top
R39  32.28,13.31 0 top
R40  49.25,30.94 0 top
R43  38.35,21.08 0 top
R44  38.33,19.61 0 top
RST  12.04,2.54 270 top
U1  50.93,53.85 270 top
U2  25.17,39.81 270 top
U3  48.79,20.42 0 top
U4  16.18,40.94 0 bottom
U5  17.32,16.51 180 top
U6  29.06,52.63 90 top
U10  7.9,48.08 180 top
U$1  [ELECROW-NEW]  42.42,38.99 0 bottom
U$5  73.88,49.63 0 top
U$8  73.88,34.37 0 top
U$10  73.88,19.05 0 top
U$12  73.88,3.81 0 top
VOUT  90.88,58.39 270 top
VOUT1  90.88,43.15 270 top
VOUT2  90.88,27.94 270 top
VOUT3  90.88,12.7 270 top
Y2  46.15,11.94 180 top

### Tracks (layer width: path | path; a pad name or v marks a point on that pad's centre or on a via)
3V3  (via drill 0.3)
  Top 0.305: U10.2 8.22,49.53 v8.69,49.07 | v10.74,34.37 10.74,30.2 13.54,27.41 13.54,24.31 v13.59,24.26
  Bottom 0.305: v13.59,24.26 13.59,19.76 16.23,17.12 33.83,17.12 34.7,17.98 34.7,20.19 39.37,24.87 42.82,24.87 48.46,19.23 48.84,19.23 49.55,18.52 49.55,4.22 J12.1 | v8.69,49.07 8.53,48.92 8.53,48.41 8.18,48.06 8.18,38.84 10.74,36.27 v10.74,34.37
5V  (via drill 0.3, 0.41, 0.61)  (1 unrouted)
  Top 0.254: 59.69,10.16 D12.C
  Top 0.305: 25.91,14.91 C21.1 | 25.91,16.31 C16.1 | v20.75,50.7 U6.14 | v9.8,49.68 9.7,49.58 9.7,48.74 8.87,47.91 U10.8 8.87,44.74 8.48,44.35 3.71,44.35 3.06,43.7 Q2.2 2.44,41.43 | U3.24 55.5,17.22 57.2,15.52 57.2,14.76 58.12,13.84 | U3.14 46.39,13.7 v46.38,13.69 | D6.+ 52.65,38.91 | 60.05,34.39 60.07,34.42 | 52.81,26.23 U3.34 52.79,26.86 v53.57,27.64 | 55.55,32.49 55.55,29.62 v55.52,29.59 | 18.41,25.88 C9.2 18.11,25.88 | 1.65,38.2 v1.63,38.18 | v45.26,29.64 45.26,27.74 44.83,27.3 44.83,26.26 U3.44
  Top 0.406: R24.1 R26.1 68.2,48.72 | R30.1 R29.1 66.93,33.5 | D8.C 60.2,36.33 | D10.C 59.94,21.34 61.09,21.34 | R37.1 R38.1 | R33.1 R34.1 | D12.C | 60.58,20.57 59.94,21.21 D10.C | v59.82,22.45 59.82,21.34 D10.C | 62.74,16.89 62.87,17.02
  Top 0.61: D3.C 60.15,47.8 61.21,46.74 62.1,46.74 | 62.1,46.74 67.31,46.74 68.2,47.62 68.2,48.72 | D8.C 60.05,34.39 | 60.05,34.39 60.05,33.3 61.47,31.88 v63.63,31.88 66.22,31.88 66.93,32.59 66.93,33.5 | 60.2,36.33 v62.1,38.23 | v62.1,45.09 62.1,46.74 | R37.1 66.68,4.45 68.12,5.89 68.12,7.7 65.79,10.03 D12.C 59.94,11.94 62.74,14.73 62.74,16.89 | R33.1 66.93,17.78 66.17,17.02 62.87,17.02 62.23,17.02 61.34,17.91 61.34,18.8 60.58,19.56 60.58,20.57 | v63.63,23.37 62.48,23.37 61.72,22.61 61.72,21.97 61.09,21.34 | C23.1 25.91,14.91 v25.91,14.94 25.91,16.31 | C16.1 D2.+ | U5.TER v17.32,14.91 U5.2 | C26.1 C23.1 | v36.07,11.68 37.74,11.68 v38.23,12.17 | v42.24,7.21 v45.87,7.21 52.02,7.21 52.43,7.62 58.17,7.62 | 59.69,10.16 59.69,8.28 59.03,7.62 58.17,7.62 | 52.65,38.91 54.61,36.96 54.61,33.43 55.55,32.49 57.15,32.49 59.05,34.39 60.05,34.39 | C11.+ 18.41,25.88 | 11.33,35.81 7.34,39.8 v6.33,39.8 | 2.44,41.43 1.65,40.64 1.65,38.2 | 18.11,25.88 17.5,25.88 16.64,26.75 16.64,31.6 | v29.34,11.66 29.08,11.66 27.25,13.49 C23.1 | 58.12,13.84 58.12,7.67 58.17,7.62
  Top 0.66: U5.2 17.32,23.27 C11.+ | 16.64,31.6 12.42,35.81 11.33,35.81
  Bottom 0.305: 59.79,22.48 59.84,22.43 | 36.04,11.66 v36.07,11.68 | v45.87,7.21 45.87,8.23 47.09,9.45 47.09,12.98 v46.38,13.69 | v53.57,27.64 53.59,27.64 53.59,27.69 54.86,28.96 | v20.75,50.7 20.75,51.05 19.99,51.82 11.94,51.82 v9.8,49.68 | v45.26,29.64 54.18,29.64 54.86,28.96 | 54.86,28.96 55.5,29.59 v55.52,29.59
  Bottom 0.61: v62.1,38.23 v62.1,45.09 | v63.63,23.37 v63.63,31.88 | v25.91,14.94 v17.32,14.91 16.92,14.5 16.92,7.9 15.11,6.1 14.4,6.81 ICSP.6 16.99,4.19 J7.1 | v29.34,11.66 36.04,11.66 | v38.23,12.17 39.67,12.17 42.01,9.83 42.01,7.44 v42.24,7.21 | v6.33,39.8 6.33,39.27 5.23,38.18 v1.63,38.18
+5V
  Top 0.305: D1.+ 32.87,19.15 33.05,18.97 33.05,16.28 R7.2
A0  (via drill 0.3)
  Top 0.305: R40.2 51.19,29.76 U3.36 51.19,18.12 v51.21,18.11
  Bottom 0.305: J8.1 31.6,1.55 51.03,1.55 52.27,2.79 52.27,6.15 51.21,7.21 v51.21,18.11
A1  (via drill 0.3)
  Top 0.305: J8.2 35.74,4.19 38.51,6.96 v38.89,6.96 39.95,6.96 41.3,8.31 v47.04,8.31 | 38.86,10.92 38.86,10.95 | 38.86,10.95 v38.86,10.97 | 38.86,10.95 39.37,11.46 39.37,12.65 38,14.02 34.21,14.02 33.5,13.31 R39.2 | U3.37 50.39,24.31 50.16,24.08 50.16,20.34 47.32,17.5 v47.32,16.89
  Bottom 0.305: v47.32,16.89 47.32,16.87 47.98,16.2 47.98,9.25 v47.04,8.31 | v38.86,10.97 38.86,6.99 v38.89,6.96
A2  (via drill 0.3)
  Top 0.305: U3.38 49.59,24.55 46.18,21.13 v46.18,20.04
  Bottom 0.305: v46.18,20.04 44.48,20.04 44.25,19.81 44.25,7.21 41.22,4.19 J9.1
A3  (via drill 0.3)
  Top 0.305: U3.39 48.79,24.74 44.98,20.93 45.01,20.9 45.01,18.95 v45.06,18.9
  Bottom 0.305: v45.06,18.9 45.06,6.88 44.24,6.07 J9.2
AREF
  Top 0.305: U3.42 46.39,30.32 C14.1
D2  (via drill 0.3)
  Top 0.305: U3.19 50.39,13.84 50.95,13.28 53.49,13.28 v54.41,12.37 | v73.2,54.3 67.84,54.3 v66.73,55.42 | R20.2 v64.52,57.68
  Top 0.406: R20.2 R14.1
  Bottom 0.305: v54.41,12.37 54.41,7.01 55.85,5.56 60.58,5.56 63.04,3.1 70.1,3.1 73.33,6.33 73.33,12.5 74.73,13.89 74.73,15.85 73.97,16.61 73.97,53.54 v73.2,54.3 | v66.73,55.42 65.91,55.42 64.52,56.82 R20.2 64.54,57.68 v64.52,57.68
D3  (via drill 0.3, 0.41)
  Top 0.305: U3.18 49.59,13.55 50.49,12.65 52.3,12.65 53.64,11.3 v56.39,11.3 | v56.39,6.43 56.39,5.05 59.36,2.08 70.18,2.08 73.69,5.59 73.69,22.15 72.26,23.57 v68.61,23.57
  Top 0.406: R27.1 R28.2 v60.58,42.16
  Bottom 0.305: v68.61,23.57 68.61,21.74 66.88,20.02 62.69,20.02 62.15,20.55 62.15,35.36 60.58,36.93 v60.58,42.16 | v56.39,6.43 56.39,6.81 55.45,7.75 55.45,10.36 v56.39,11.3
D4  (via drill 0.3, 0.41)
  Top 0.305: U3.25 53.23,18.02 v52.96,18.29
  Top 0.406: R31.1 R32.2 v59.31,27.05
  Bottom 0.305: v52.96,18.29 52.96,19.18 54,20.22 54.03,20.22 56.54,22.73 57.17,22.73 57.78,23.34 57.78,25.53 v59.31,27.05
D5  (via drill 0.3, 0.41)
  Top 0.305: U3.31 57.27,22.82 57.91,22.17 57.91,15.19 v59.77,13.34
  Top 0.406: R36.2 R35.1 v62.87,13.34
  Bottom 0.305: v59.77,13.34 v62.87,13.34
D6  (via drill 0.3)
  Top 0.305: U3.27 55.41,19.62 v55.75,19.96 | v38.91,54.33 v37.24,52.65 | v33.07,55.98 33.07,57.53 35.2,59.66 35.2,61.57 J1.2
  Bottom 0.305: v55.75,19.96 61.01,19.96 61.49,20.45 61.49,35.03 59.99,36.52 59.99,41.35 59.36,41.99 59.36,49.73 53.67,55.42 40.01,55.42 v38.91,54.33 | v37.24,52.65 34.16,52.65 33.05,53.77 33.05,55.96 v33.07,55.98
D7  (via drill 0.3)
  Top 0.305: v26.82,37.47 26.82,43.56 v25.17,45.21 | v26.04,57.4 26.06,57.4 30.23,61.57 J1.1 | U3.1 42.99,25.46 42.16,26.29 v42.16,27.05
  Bottom 0.305: v26.82,37.47 26.85,37.44 26.85,32.66 27.28,32.23 32.82,32.23 33.71,33.12 34.67,33.12 35.18,32.61 40.41,32.61 42.16,30.86 v42.16,27.05 | v25.17,45.21 25.17,56.54 v26.04,57.4
D+1  (via drill 0.3)
  Top 0.305: v36.02,15.49 36.07,18.11 R44.1 | J11.3 6.33,10.41 6.63,10.11 18.49,10.11 18.62,9.98 v18.62,9.96 | v36.02,12.9 35.76,12.9 32.97,10.11 v25.48,10.11
  Bottom 0.305: v18.62,9.96 25.32,9.96 v25.48,10.11 | v36.02,12.9 36.09,12.98 36.09,15.47 v36.02,15.49
D-1  (via drill 0.3)
  Top 0.305: v34.39,12.65 32.82,10.95 v24.49,10.95 | v34.37,15.54 34.37,19.23 36.2,21.06 37.69,21.06 37.72,21.08 R43.1 | J11.2 6.64,11.06 7.01,10.69 19.71,10.69 v20.04,10.82
  Bottom 0.305: v34.39,12.65 34.39,15.52 v34.37,15.54 | v20.04,10.82 24.31,10.77 v24.49,10.95
DTR_5V  (via drill 0.3)
  Top 0.305: U6.11 v27.3,52.63 | U3.28 v52.96,20.4
  Bottom 0.305: v52.96,20.4 51.23,20.42 49.99,21.67 47.24,21.67 45.8,23.11 45.8,23.16 43.31,25.65 39.14,25.65 34.42,20.93 34.42,20.9 33.88,20.37 29.64,20.37 27.3,22.71 25.86,22.71 24,24.56 24,29.79 20.65,33.15 20.65,40.36 22.35,42.06 24.28,42.06 27.3,45.09 v27.3,52.63
GATE
  Top 0.305: Q2.1 4.96,43.14 5.38,43.56 9.07,43.56 11.56,46.05 11.56,51.92 11.1,52.38 10.34,52.38 9.65,51.69 9.12,51.69 8.87,51.45 U10.1
GND  (via drill 0.3, 0.41)
  other vias: 62.74,54.36 65.79,15.11 66.04,57.66 68.58,11.81 37.31,46 40.34,46.02 39.12,18.08 37.36,17.35 44.2,21.26 43,11.4 46.46,16.21 46.15,11.89 45.8,9.19 41.73,20.65 48.79,20.42 54.61,15.32 30.33,38.35 27.94,18.85 13.31,13.34 59.23,19.05 58.98,3.94 35.64,10.29 48.44,31.01 52.22,27.64 19.76,26.04 18.24,27.58 62.43,8.36 66.09,11.79 65.99,7.95 69.34,7.77 65.05,50.52 32.92,47.62 21.84,37.36 23.9,52.35 16.03,54.74 14.53,47.32 10.34,47.73 9.86,50.9 35.23,16.51 32.33,22.05 35.81,19.56 37.85,22.15 40.28,24.13 31.55,29.84 29.31,29.95 25.88,34.42 15.09,49.76
  pour Top: 2.31,66.09 75.13,66.09 75.13,-0.1 0.38,-0.1 -0.13,0.41 -0.13,65.46 -0.09,65.61 -0.07,65.67 -0.04,65.76 0.01,65.84 0.07,65.93 0.34,66.12 0.41,66.15 0.52,66.16 0.58,66.17 0.62,66.17 2.31,66.17
  pour Bottom: 2.34,66.14 74.6,66.14 75.11,65.63 75.11,-0.13 0.36,-0.13 -0.15,0.38 -0.13,65.63 0.37,66.14 2.29,66.19
GSM_ANT
  Top 0.305: C24.2 30.1,28.94 R25.2 30.04,31.77 U2.32
IO9  (via drill 0.3)
  Top 0.305: U3.29 53.45,21.22 52.96,21.72 v52.96,22.35 | v44.2,28.45 42.04,28.45 v40.77,27.18 | v32.89,23.37 32.89,24.16 R3.1
  Bottom 0.305: v52.96,22.35 52.96,23.62 48.13,28.45 v44.2,28.45 | v40.77,27.18 36.58,27.18 35.81,26.42 35.81,24.26 34.54,22.99 33.27,22.99 v32.89,23.37
IO10  (via drill 0.3, 0.41)
  Top 0.305: v72.97,53.01 67.82,53.01 v66.7,54.13 | U3.30 56.74,22.02 57.15,21.61 57.15,17.78 v56.95,17.58
  Bottom 0.305: 62.1,11.56 59,11.56 56.95,13.61 v56.95,17.58 | v66.7,54.13 65.3,54.13 62.46,56.97 29.69,56.97 J3.2
  Bottom 0.406: v72.97,53.01 72.9,16.38 73.91,15.37 73.91,14.48 72.9,13.46 71.37,13.46 70.61,12.7 70.1,13.21 65.28,13.21 63.63,11.56 62.1,11.56
IO11  (via drill 0.3, 0.41)
  Top 0.305: U3.12 44.79,13.73 44.04,12.98 44.04,10.77 44.88,9.93 v56.57,9.93
  Top 0.406: v64.9,61.09 v71.76,61.09 | v71.37,21.34 71.37,13.97 72.26,13.08 v72.26,11.56
  Bottom 0.305: 64.77,60.96 59.82,60.96 59.13,61.65 38.07,61.65 35.76,63.96 20.73,63.96 20.07,63.3 J3.1 | v56.57,9.93 71.32,9.93 72.26,10.87 v72.26,11.56
  Bottom 0.406: 64.77,60.96 v64.9,61.09 | v71.76,61.09 71.76,21.72 v71.37,21.34
IO12  (via drill 0.3)
  Top 0.305: v55.6,18.82 U3.26 | 54.56,18.8 U3.26 | U3.26
  Bottom 0.254: 68.58,63.5 68.64,63.56
  Bottom 0.305: 68.71,63.5 70.61,61.59 70.61,31.62 70.1,31.11 70.1,16.38 69.22,15.49 68.07,15.49 66.55,17.02 62.1,17.02 61.47,16.38 59.46,16.38 57.02,18.82 v55.6,18.82 | 68.58,63.5 47.04,63.5 45.64,64.9 17.02,64.9 14.88,62.76 14.88,61.62 J6.2
  Bottom 0.406: 68.58,63.5 68.71,63.5
IO13  (via drill 0.3, 0.41)
  Top 0.305: v67.18,30.48 59.66,30.48 57.68,28.5 57.68,24.03 57.28,23.62 U3.32 | J6.1 9.91,63.07 11.63,64.8 30.79,64.8 32.99,62.59 32.99,60.38 v33.68,59.69
  Bottom 0.305: v33.68,59.69 66.04,59.69 68.07,57.66 68.07,31.37 v67.18,30.48
MISO  (via drill 0.3)  (1 unrouted)
  Top 0.305: ICSP.1 23.42,8.84 24,8.26 39.65,8.26 41.6,10.21 v41.6,12.24 | U3.11 42.08,16.42 v41.6,15.54
  Bottom 0.305: 41.53,12.27 41.53,12.24 | v41.6,15.54 v41.6,12.24
MOSI  (via drill 0.3)
  Top 0.305: ICSP.5 12.34,6.15 13.31,5.18 14.86,5.18 17.68,8 23.27,8 23.72,7.54 37.08,7.54 v37.11,7.52 | v37.11,15.47 40.01,15.47 41.76,17.22 U3.10
  Bottom 0.305: v37.11,7.52 v37.11,15.47
N$1  (via drill 0.3)
  Top 0.305: R19.2 10.95,43.33 v12.88,45.26
  Bottom 0.305: v12.88,45.26 14.1,45.26 16.09,47.26 U4.7
N$2
  Top 0.406: R6.2 R4.1
  Top 0.61: U1.5 54.23,53.14 54.46,53.37 56.77,53.37 57.58,54.18 57.63,54.18 57.78,54.33 57.78,58.01 58.83,59.05 R4.1
N$3
  Top 0.406: R14.2 70.23,59.18 70.46,59.41 | 70.46,59.41 70.48,59.44 | Q3.1 70.46,59.41
N$4  (via drill 0.61)
  Top 0.305: 13.18,33.1 v13.16,33.12 | 28.8,36.09 v28.83,36.12
  Top 0.61: v13.18,29.84 13.18,33.1 | v49.76,36.12 50.34,36.12 50.82,35.64 D5.+ | 28.8,36.09 v25.98,36.09 | v22,36.12 19.23,36.12 v19.18,36.07
  Bottom 0.61: v13.18,29.84 12.45,29.11 12.45,19.3 11.56,18.41 J4.+ | v28.83,36.12 v49.76,36.12 | v13.16,33.12 16.23,33.12 v19.18,36.07 | v25.98,36.09 22.53,36.09 v22,36.12
N$5  (via drill 0.3)
  Top 0.305: R18.1 6.31,41.26 5.99,41.58 5.99,42.47 6.38,42.85 9.37,42.85 12.95,46.43 v12.95,46.46
  Bottom 0.305: U4.3 13.95,48.52 12.95,47.52 v12.95,46.46
N$6  (via drill 0.3)
  Top 0.305: 10.13,39.85 v9.65,39.85 9.66,39.84 R17.1
  Bottom 0.305: v9.65,39.85 8.97,40.54 8.97,43.64 12.01,46.69 12.01,49.23 13.64,50.85 18.44,50.85 19.76,49.53 19.76,46.97 18.78,45.98 U4.2
N$7
  Top 0.406: R13.2 4.22,54.13 3.17,53.09 3.17,51.46 NETLIGHT.+
N$8
  Top 0.406: D7.- 62.31,50.76 U$5.IN- 64.39,52.83 64.39,56.39 | Q3.3 72.52,57.4 71.5,56.39 64.39,56.39 | 64.39,56.39 61.09,56.39 60.19,55.49 D3.A
N$9
  Top 0.305: L.+ R12.2 4.8,47.02
N$10
  Top 0.406: R31.2 69.34,28.7 Q6.1
N$11
  Top 0.305: U10.7 U10.6 7.57,47.09 6.12,48.54 R12.1
N$12
  Top 0.406: D7.+ R24.2
N$13
  Top 0.406: D11.- 62.48,20.35 U$10.IN- 63.75,21.59 65.79,23.62 65.79,25.27 | D10.A 65.79,25.27 | 65.79,25.27 70.1,25.27 71.63,26.8 Q6.3 | 65.79,25.27
N$14  (via drill 0.3)
  Top 0.305: R23.2 7.57,51.34 U10.3 v7.57,49.26 v7.57,49.25 | v22.91,29.11 22.91,28.5 22.88,28.47 22.91,28.45 R22.2
  Bottom 0.305: v22.91,29.11 22.22,29.79 16.03,29.79 14.58,31.24 12.7,31.24 11.07,32.87 6.66,32.87 5.69,33.83 5.69,36.73 7.57,38.61 v7.57,49.25
N$15
  Top 0.305: R8.2 D1.-
N$16
  Top 0.305: R21.2 25.86,20.85 Q4.3
N$17
  Top 0.305: D2.- R21.1
N$18
  Top 0.305: Q4.1 30.45,22.91 31.27,23.72 31.27,26.19 32.03,26.95 35.36,26.95 35.81,26.49 R16.1 R15.2
N$19
  Top 0.406: R26.2 69.67,50.85 68.33,52.2 66.28,52.2 U$5.IN+
N$20
  Top 1.778: U$5.L2 84.04,56.94 arc45 83.67,57.84 C8.2 arc45 83.54,58.4 VOUT.1
N$21
  Top 1.778: C8.1 76.79,55.99 arc45 76.42,55.09 U$5.L1 79.71,48.89 arc45 80.6,48.51 89.03,48.51 90.51,49.99 arc45 90.88,50.89 VOUT.2
N$22
  Top 0.406: R27.2 68.05,43.81 Q5.1
N$23
  Top 0.406: D9.- 62.43,35.62 U$8.IN- 63.72,40.22 63.88,40.38 | D8.A 63.88,40.38 | 63.88,40.38 68.83,40.38 70.1,41.66 Q5.3
N$24
  Top 0.406: D9.+ R29.2
N$25
  Top 0.305: C25.2 29.08,28.94 R25.1 28.89,29.26 GSM.D
N$26
  Top 0.406: R30.2 69.93,36.25 69.22,36.96 66.31,36.96 U$8.IN+
N$27
  Top 1.778: U$8.L2 84.04,41.42 arc45 83.67,42.32 C12.2 arc45 83.05,43.16 VOUT1.1
N$28
  Top 1.778: C12.1 76.79,40.72 arc45 76.42,39.83 U$8.L1 79.55,33.77 arc45 80.45,33.4 88.01,33.4 90.51,35.9 arc45 90.88,36.8 VOUT1.2
N$29
  Top 0.406: D11.+ R33.2
N$30
  Top 0.406: U$10.IN+ 68.33,21.59 69.98,19.94 R34.2
N$31
  Top 1.778: U$10.L2 84.04,26.3 arc45 83.67,27.2 C13.2 arc45 83.29,27.94 VOUT2.1
N$32
  Top 1.778: C13.1 76.79,25.61 arc45 76.42,24.71 U$10.L1 79.48,18.53 arc45 80.38,18.16 88.01,18.16 90.51,20.66 arc45 90.88,21.56 VOUT2.2
N$33
  Top 0.406: R35.2 68.33,13.34 Q7.1
N$34  (via drill 0.41)
  Top 0.406: D12.A 59.94,4.83 61.21,3.56 D13.- | 62.36,3.56 D13.- | D13.- 62.23,4.86 U$12.IN- 63.72,7.71 v64.52,8.51 | v70.61,8.89 Q7.3
  Bottom 0.406: v70.61,8.89 64.9,8.89 v64.52,8.51
N$35
  Top 0.406: D13.+ R37.2
N$36  (via drill 0.3)
  Top 0.305: R3.2 R2.1 v34.39,25.68 | v38.86,31.5 38.91,31.55 Q1.1 38.86,31.55
  Bottom 0.305: v38.86,31.5 38.3,31.5 34.39,27.58 v34.39,25.68
N$37  (via drill 0.41)
  Top 0.406: v69.6,5.46 R38.2
  Bottom 0.406: U$12.IN+ 68.71,6.35 v69.6,5.46
N$38
  Top 1.778: U$12.L2 84.04,11.19 arc45 83.67,12.09 82.8,12.95 C17.2 arc45 83.29,12.7 VOUT3.1
N$39
  Top 1.778: C17.1 76.79,10.37 arc45 76.42,9.47 U$12.L1 79.1,3.67 arc45 79.99,3.3 87.5,3.3 90.51,6.31 arc45 90.88,7.21 VOUT3.2
N$53
  Top 0.305: 40.32,47.46 PWR.-
  Top 0.61: R1.1 40.32,47.46
NETLIGHT
  Top 0.305: U2.41 32.97,43.1 32.23,43.84 32.23,45.16 35.38,48.31 35.38,53.03 35.14,53.28 U6.5
NETLIGHT_5V
  Top 0.305: U6.10 12.96,53.28 12.12,54.13 R13.1
PWR_IN  (via drill 0.3, 0.61)
  Top 0.305: U5.3 15.04,24.28 v15.01,24.31 | v19.81,28.52 C7.2 R22.1 21.39,29.21 20.65,29.95 17.83,29.95 17.55,30.23 17.55,34.37 18.21,35.03 18.21,36.8 20.14,38.73 v22.25,38.73 | v37.8,49.61 C10.+ | v29.11,40.21 29.11,44.83 v29.79,45.52
  Top 0.61: 56.46,35.23 D5.- 56.46,35.81 D4.+ v56.46,40.84 | v39.8,49.61 v37.8,49.61
  Bottom 0.305: v15.01,24.31 15.01,27.18 16.97,29.13 19.2,29.13 v19.81,28.52 | v22.25,38.73 27.63,38.73 v29.11,40.21 | v29.79,45.52 33.53,45.52 37.62,49.61 v37.8,49.61
  Bottom 0.61: v56.46,40.84 56.46,48.9 52.45,52.91 52.43,52.91 51.77,53.57 44.65,53.57 40.69,49.61 v39.8,49.61
PWRKEY  (via drill 0.3)  (1 unrouted)
  Top 0.305: U2.39 35.4,40.91 v35.41,40.92 | Q1.3 39.78,34.24 40.08,34.54 v44.3,34.54 | v46.89,35 46.89,36.3 v46.13,37.52 | PON/POFF.P$2 42.75,63.37 38.1,58.73 35.56,58.73 35.03,58.19 v35.03,55.58 | v39.57,40.89 v39.57,43.61
  Bottom 0.305: v44.3,34.54 46.43,34.54 v46.89,35 | v46.13,37.52 39.98,37.52 39.57,37.9 v39.57,40.89 39.55,40.89 | 39.55,40.92 v35.41,40.92 | v35.03,55.58 35.66,54.94 36.5,54.94 39.57,51.87 39.57,51.59 38.94,50.95 38.91,50.95 38.84,50.88 38.84,45.39 39.57,44.65 v39.57,43.61 39.57,43.51
RD+
  Top 0.305: U3.4 42.06,22.02 | R44.2 40.16,19.61 40.62,20.07 40.62,20.88 41.76,22.02 42.06,22.02 | 42.06,22.02
RD-
  Top 0.305: U3.3 41.74,22.82 40.01,21.08 R43.2
RESET  (via drill 0.3)
  Top 0.305: RST.P$1 13.21,2.54 11.07,4.67 7.98,4.67 7.57,5.08 7.57,7.42 8.99,8.84 ICSP.3 | v29.84,14.73 R8.1 R7.1 33.1,14.71 43.46,14.71 44.5,15.75 45.26,15.75 45.59,15.42 U3.13
  Bottom 0.305: RST.P$1 26.06,2.54 26.7,3.17 26.7,11.58 v29.84,14.73
RXD_5V  (via drill 0.3)
  Top 0.305: U6.12 26.68,51.98 27.25,51.41 v28.5,51.41 | U3.21 51.99,23.52 54.89,26.42 54.89,28.09 49.89,33.1 45.74,33.1 45.29,33.55 45.29,36.35 44.68,36.96 v44.68,40.82
  Bottom 0.305: v28.5,51.41 28.5,44.93 31.42,42.01 43.48,42.01 v44.68,40.82
SCK  (via drill 0.3)
  Top 0.305: U3.9 42.05,18.02 v42.01,18.06
  Bottom 0.305: ICSP.2 12.34,15.04 13.13,15.82 33.33,15.82 36.96,19.46 39.6,19.46 40.13,18.92 40.13,18.34 40.41,18.06 v42.01,18.06
SIM_CLK
  Top 0.305: U2.16 12.83,40.91 R18.2
SIM_DATA
  Top 0.305: U2.15 14.23,42.01 13.54,42.7 12.47,42.7 | 12.47,42.7 12.37,42.7 12.34,42.72 | R19.1 12.47,42.7
SIM_RST
  Top 0.305: U2.17 12.5,39.81 R17.2
SIM_VDD  (via drill 0.3)
  Top 0.305: U2.18 15.47,38.71 14.86,38.1 14.07,38.1 14.02,38.05 v14.02,38.18 13.81,38.39 C20.1
  Bottom 0.305: U4.1 12.51,43.45 12.07,43 12.07,38.71 12.6,38.18 v14.02,38.18
STATUS  (via drill 0.3)
  Top 0.305: U2.42 34.09,44.2 36.63,44.2 37.59,43.23 v37.59,39.67 | R15.1 39.01,28.22 39.52,28.73 39.52,29.34 38.53,30.33 34.54,30.33 v34.29,30.58 | v23.49,34.82 v23.49,40.66
  Bottom 0.305: v23.49,34.82 23.49,33.91 24.38,33.02 24.38,32.99 26.67,30.71 34.16,30.71 v34.29,30.58 | v23.49,40.66 27.3,40.66 28.3,41.66 30.18,41.66 32.16,39.67 v37.59,39.67
TXD_5V  (via drill 0.3)
  Top 0.305: U6.13 23.22,51.33 v22.5,52.05 | U3.20 51.19,16.34 50.75,16.79 48.79,16.79 v48.72,16.87 | v47.02,18.54 47.02,20.85 v48.77,22.61 | v24.61,34.37 24.61,43.64 v22.5,45.74 | v34.57,32.05 34.57,33.96 v34.98,34.37
  Bottom 0.305: v48.72,16.87 48.69,16.87 v47.02,18.54 | v22.5,45.74 v22.5,52.05 | v34.98,34.37 35.92,35.31 40.64,35.31 43.05,32.89 43.05,26.92 47.37,22.61 v48.77,22.61 | v24.61,34.37 24.61,33.81 26.82,31.6 34.11,31.6 v34.57,32.05
UART_DTR
  Top 0.305: U2.6 25.72,49.67 25.86,49.81 28.19,49.81 31.01,52.63 U6.4
UART_RXD
  Top 0.305: U6.3 31.43,51.98 30.12,50.67 U2.2
UART_TXD
  Top 0.305: U6.2 33.02,51.33 33.55,50.8 33.55,49.38 33.1,48.92 31.42,48.92 31.22,48.72 U2.1
UCAP  (via drill 0.3)
  Top 0.305: U3.6 43.87,20.42 44.22,20.07 44.22,16.84 44.2,16.82 44.2,16.2 43.48,15.49 v42.8,15.49 | v39.09,16.54 C15.1 | v39.34,13.97 v42.8,13.97
  Bottom 0.305: v42.8,15.49 v42.8,13.97 | v39.09,16.54 39.12,15.72 39.12,14.2 v39.34,13.97
VBAT
  Top 0.254: 60.96,62.23 C5.2
  Top 0.406: R5.2 C5.2 R4.2 | U2.34 U2.35
  Top 0.61: U1.4 52.58,53.52 53.57,54.51 56.03,54.51 56.57,55.04 56.57,58.65 58.52,60.6 58.55,60.58 R4.2 | U2.35 41.84,36.51 42.52,37.19 C4.+
  Top 1.676: C4.+ 42.52,40.01 42.52,43.84 45.41,46.74 52.02,46.74 52.58,47.3 U1.4
VDD_EXT  (via drill 0.3)
  Top 0.305: U6.8 28.78,54.58 v29.74,53.62 | v31.24,49.96 32.77,49.96 32.92,50.11 32.92,50.39 32.63,50.68 U6.1 | U2.40 31.68,42.01 31.27,42.42 v31.27,46.25
  Bottom 0.305: v29.74,53.62 29.74,51.46 v31.24,49.96 31.27,49.94 v31.27,46.25
VIN  (via drill 0.3)  (4 unrouted)
  Top 0.305: C1.2 41.86,46.15 | PWR.+
  Top 0.406: 47.6,50.55 47.62,50.52 | U1.1 U1.2
  Top 0.61: C2.2 38.89,45.36 39.47,44.78 41.17,44.78 41.86,45.47 C1.2 PWR.+ | v47.68,51.64 47.68,50.85 47.6,50.77 47.57,50.77 47.55,50.8 | v47.62,49.66 v48.41,49.66 48.54,49.78 49.28,49.78 v49.35,49.71 49.35,50.47 U1.2 49.45,50.72 v49.45,50.75 | v47.68,51.64 48.51,51.64 v48.54,51.66 49.4,51.66 v49.43,51.69 | v49.28,43.79 49.23,43.84 v48.41,43.84 48.36,43.79 v47.5,43.79 v47.5,42.9 | v49.3,42.85 48.41,42.85 v48.39,42.88 47.5,42.88 | v47.5,42.9 47.5,42.88 | 47.5,42.88 47.47,42.88 v47.5,42.9 | PWR.+ 41.86,51.91 42.21,52.27 C3.+ 42.85,51.64 v47.68,51.64
  Top 1.27: v49.3,42.85 52.12,42.85 D6.- D4.-
  Bottom 0.61: v48.41,49.66 v48.41,43.84
  other vias: 48.44,50.8 47.57,50.8
VRTC  (via drill 0.3)
  Top 0.305: C6.2 42.44,29.92 41.43,28.91 v40.46,28.91 | v38.35,28.91 v33.17,28.91 | v25.7,30.4 25.7,31.83 | 25.7,31.83 25.7,31.9 | U2.28 25.72,31.84 25.7,31.83
  Bottom 0.305: v40.46,28.91 v38.35,28.91 | v33.17,28.91 27.2,28.91 v25.7,30.4
VUSB  (via drill 0.3)
  Top 0.305: U3.2 | v41.33,23.62 41.81,23.62 | U3.2 v41.33,23.62 | v41.33,23.62 | C19.1 v38.99,22.68 | U3.7 42.25,19.62 v42.24,19.63 40.59,17.98 v40.59,17.14 | 40.62,13.06 40.59,13.03 v40.59,13.01 40.59,11.1 38.61,9.12 24.33,9.12 21.77,11.68 | 21.77,11.68 21.74,11.71 21.72,11.71 8.25,11.71 | 21.77,11.66 21.77,11.68
  Top 0.406: J11.1 7.31,11.71 7.32,11.71
  Top 0.61: Q2.3 4.01,38.41 5.03,37.39 5.03,24.99 6.48,23.55 6.48,14.71 8.2,12.98 8.2,11.76 8.25,11.71 7.32,11.71
  Bottom 0.305: 40.59,22.73 40.59,19.63 v42.24,19.63 | 40.59,22.73 40.59,22.89 v41.33,23.62 | v38.99,22.68 40.54,22.68 40.59,22.73 | v40.59,13.01 v40.59,17.14
XTAL3
  Top 0.305: R9.2 47.38,11.71 Y2.1 47.99,12.78 U3.16
XTAL4
  Top 0.305: U3.17 48.79,13.36 R9.1 50.44,10.9 50.04,10.49 45.36,10.49 45.15,10.7 Y2.3
(copper drawn outside any net)
  shapes: Bottom area x1, Top area x5

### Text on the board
tPlace: 13 | 12 | 11 | 10 | 7 | 6 | 5V | GND | A0 | A1 | A2 | A3 | 3V3 | GND
bPlace: SIM Card Holder | Leonardo GPRS/GSM IOT Board | v1.0 | www.elecrow.com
